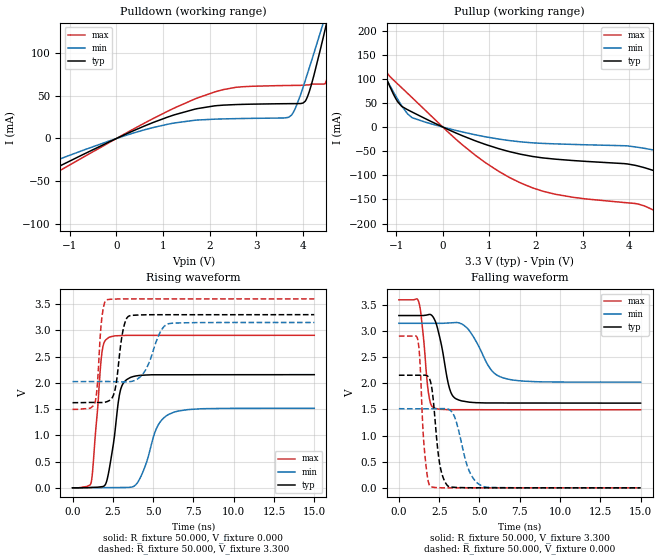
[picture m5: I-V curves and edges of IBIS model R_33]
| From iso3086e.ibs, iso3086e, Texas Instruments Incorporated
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|   R_33 MODEL
[Model]   R_33
Model_type   3-state
Polarity   Non-Inverting
Enable   Active-Low
Vmeas   = 1.50
Cref   = 15pF
|   typ   min   max
C_comp   4.19pF   4.70pF   4.47pF
|C_comp (High state)   1.86pF   1.85pF   1.86pF
[Voltage Range]   3.3   3.15   3.6
[Temperature Range]   40   125   -40
[Pullup Reference]   3.3   3.15   3.6
[Pulldown Reference]   0   0   0
[Power Clamp Reference]   3.3   3.15   3.6
[GND Clamp Reference]   0   0   0
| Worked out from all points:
|   slope of the pulldown table from 0 to 0.495 V, typ, clamps not added: 40.6 ohm
|   slope of the pullup table from 0 to 0.495 V, typ, clamps not added: 23.7 ohm
|   falling waveform, R_fixture 50.000, V_fixture 3.300: 20-80 % time 625ps typ, 1.2ns min, 373ps max; typ from 3.3 V to 1.62 V
|   rising waveform, R_fixture 50.000, V_fixture 0.000: 20-80 % time 566ps typ, 979ps min, 429ps max; typ from 0 V to 2.16 V
|   rising waveform, R_fixture 50.000, V_fixture 3.300: 20-80 % time 419ps typ, 841ps min, 273ps max; typ from 1.62 V to 3.3 V
|   falling waveform, R_fixture 50.000, V_fixture 0.000: 20-80 % time 430ps typ, 782ps min, 305ps max; typ from 2.16 V to 0 V
[Pulldown]
|   Voltage   I(typ)   I(min)   I(max)
-3.3V     -89.75mA   -69.39mA   -103.5mA
-706.2mV  -18.6mA    -13.69mA   -21.89mA
1.11V     25.36mA    16.83mA    32.32mA
2.293V    39.16mA    22.99mA    57.43mA
3.689V    40.88mA    24.87mA    62.26mA
3.843V    40.94mA    36.33mA    62.32mA
4.066V    45.45mA    71.14mA    62.81mA
4.184V    64.23mA    91.58mA    63.85mA
4.392V    109.2mA    128.3mA    63.89mA
4.486V    131mA      145.3mA    65.83mA
4.734V    189.8mA    190.4mA    132mA
6.6V      650.9mA    540.4mA    767.3mA
[Pullup]
|   Voltage   I(typ)   I(min)   I(max)
-3.3V     612.5mA    489.8mA    809.7mA
-1.825V   246.9mA    211.8mA    304.5mA
-1.558V   182.1mA    162.4mA    215.7mA
-1.196V   97.48mA    96.98mA    112.8mA
-968.6mV  52.67mA    57.95mA    89.47mA
-666.6mV  31.61mA    20.13mA    61.82mA
684.7mV   -28.01mA   -15.78mA   -57.4mA
1.675V    -56.4mA    -30.68mA   -116.1mA
2.417V    -66.53mA   -34.84mA   -139.3mA
4.17V     -80.28mA   -41.73mA   -159.1mA
5.174V    -112.2mA   -60.77mA   -206mA
6.6V      -169.1mA   -95.93mA   -291mA
[Ramp]
R_load = 50
|   typ   min   max
dV/dt_r   1.29384/5.65785e-010  0.908858/9.79654e-010   1.74337/4.28854e-010
dV/dt_f   1.0206/6.23606e-010  0.675573/1.19616e-009   1.263/3.72554e-010
[Falling Waveform]
R_fixture = 50.000
V_fixture = 3.300
V_fixture_min = 3.150
V_fixture_max = 3.600
C_fixture = 0.000
|  time   V(typ)   V(min)   V(max)
0s        3.299V     3.15V      3.6V
1.233ns   3.299V     3.15V      3.558V
1.386ns   3.299V     3.15V      3.283V
1.827ns   3.316V     3.15V      1.835V
2.173ns   3.245V     3.15V      1.532V
2.599ns   2.794V     3.15V      1.503V
3.136ns   1.908V     3.158V     1.496V
3.714ns   1.682V     3.16V      1.496V
6.417ns   1.625V     2.111V     1.495V
15ns      1.622V     2.024V     1.495V
[Rising Waveform]
R_fixture = 50.000
V_fixture = 0.000
V_fixture_min = 0.000
V_fixture_max = 0.000
C_fixture = 0.000
|  time   V(typ)   V(min)   V(max)
0s        2.723nV    15.31nV    2.666nV
1.166ns   7.941mV    2.366mV    115.2mV
1.827ns   22.89mV    3.706mV    2.584V
2.225ns   269.2mV    4.513mV    2.86V
2.983ns   1.874V     6.051mV    2.9V
3.553ns   2.097V     10.4mV     2.905V
4.139ns   2.141V     153.6mV    2.905V
5.193ns   2.154V     1.123V     2.905V
5.977ns   2.154V     1.401V     2.905V
15ns      2.156V     1.515V     2.906V
[Rising Waveform]
R_fixture = 50.000
V_fixture = 3.300
V_fixture_min = 3.150
V_fixture_max = 3.600
C_fixture = 0.000
|  time   V(typ)   V(min)   V(max)
0s        1.622V     2.024V     1.495V
1.386ns   1.627V     2.025V     1.617V
1.827ns   1.625V     2.026V     3.259V
2.12ns    1.641V     2.026V     3.582V
2.599ns   1.822V     2.023V     3.597V
3.136ns   3.007V     2.018V     3.6V
3.553ns   3.279V     2.023V     3.6V
4.489ns   3.296V     2.223V     3.6V
5.977ns   3.298V     3.128V     3.6V
15ns      3.299V     3.15V      3.6V
[Falling Waveform]
R_fixture = 50.000
V_fixture = 0.000
V_fixture_min = 0.000
V_fixture_max = 0.000
C_fixture = 0.000
|  time   V(typ)   V(min)   V(max)
0s        2.156V     1.515V     2.906V
1.166ns   2.156V     1.514V     2.843V
1.287ns   2.156V     1.514V     2.521V
1.599ns   2.157V     1.514V     679.1mV
1.987ns   2V         1.514V     21.69mV
2.533ns   456mV      1.516V     2.208mV
3.06ns    30.84mV    1.506V     138uV
4.373ns   2.069mV    315.6mV    122.8uV
5.193ns   838.7uV    31.03mV    113.3uV
15ns      -17.17nV   145.7nV    -6.692nV
